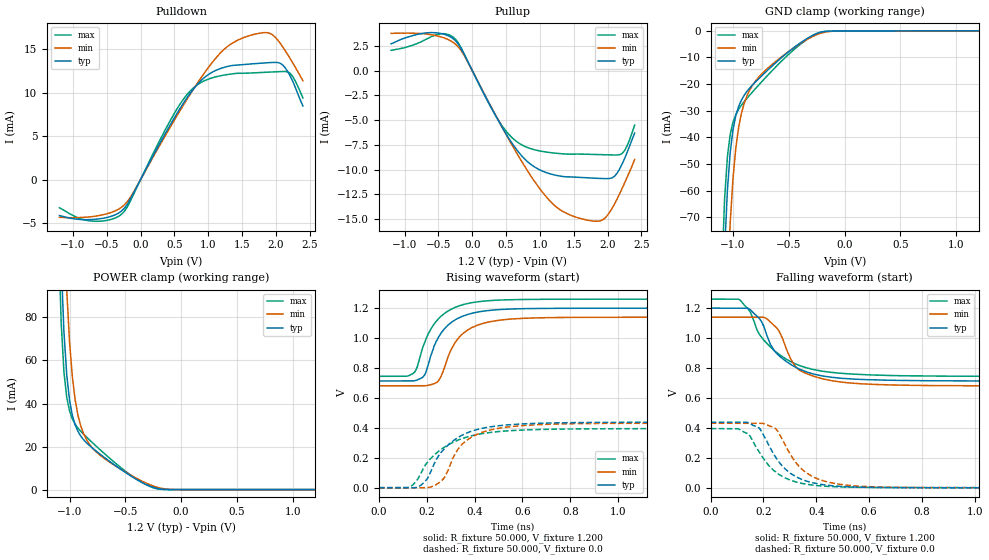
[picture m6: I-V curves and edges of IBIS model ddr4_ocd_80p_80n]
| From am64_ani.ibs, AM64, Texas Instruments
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|   Model ddr4_ocd_80p_80n
[Model] ddr4_ocd_80p_80n
Model_type I/O
Polarity   Non-Inverting
Enable   Active-High
Vinl =  0.700V
Vinh =  0.900V
Vmeas =  0.600V
C_comp   2.607pF   2.588pF   2.639pF
[Model Spec]
Vinh   0.900V   0.820V   0.980V
Vinl   0.700V   0.620V   0.780V
Vmeas   0.600V   NA   NA
[Temperature Range]   25.000   0.125k   -40.000
[Voltage Range]   1.200V   1.140V   1.260V
[Pullup Reference]   1.200V   1.140V   1.260V
[Pulldown Reference]   0.0V   0.0V   0.0V
[C Comp Corner]
C_comp   2.588pF   2.639pF   2.607pF
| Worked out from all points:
|   slope of the pulldown table from 0 to 0.18 V, typ, clamps not added: 67.6 ohm
|   slope of the pullup table from 0 to 0.18 V, typ, clamps not added: 74.1 ohm
|   GND clamp passes 1 mA (typ) near -0.25 V on its own axis
|   POWER clamp passes 1 mA (typ) near -0.25 V on its own axis
|   rising waveform, R_fixture 50.000, V_fixture 1.200: 20-80 % time 96.8ps typ, 97.8ps min, 100ps max; typ from 0.714 V to 1.2 V
|   rising waveform, R_fixture 50.000, V_fixture 0.0: 20-80 % time 136ps typ, 115ps min, 158ps max; typ from 0.002 V to 0.44 V
|   falling waveform, R_fixture 50.000, V_fixture 1.200: 20-80 % time 121ps typ, 91.9ps min, 143ps max; typ from 1.2 V to 0.714 V
|   falling waveform, R_fixture 50.000, V_fixture 0.0: 20-80 % time 110ps typ, 110ps min, 109ps max; typ from 0.44 V to 0.002 V
[Pulldown]
|Voltage   I(typ)   I(min)   I(max)
-1.2V     -4.138mA   -4.341mA   -3.244mA
-755mV    -4.611mA   -4.296mA   -4.748mA
-309mV    -3.777mA   -3.332mA   -4.155mA
-124mV    -1.85mA    -1.702mA   -2.032mA
396mV     5.718mA    5.465mA    6.181mA
693mV     9.481mA    9.32mA     9.848mA
990mV     12.02mA    12.77mA    11.53mA
1.398V    13.17mA    15.89mA    12.21mA
1.843V    13.43mA    16.92mA    12.35mA
2.066V    13.39mA    15.67mA    12.43mA
2.214V    11.88mA    13.89mA    12.21mA
2.4V      8.473mA    11.38mA    9.385mA
[Pullup]
|Voltage   I(typ)   I(min)   I(max)
-1.2V     2.716mA    3.765mA    2.056mA
-606mV    3.849mA    3.636mA    3.437mA
-421mV    3.694mA    3.326mA    3.74mA
-235mV    2.926mA    2.597mA    3.08mA
285mV     -3.787mA   -3.737mA   -3.812mA
544mV     -6.885mA   -6.995mA   -6.474mA
915mV     -9.714mA   -11.15mA   -7.988mA
1.361V    -10.72mA   -14.32mA   -8.419mA
1.955V    -10.91mA   -14.94mA   -8.5mA
2.103V    -10.67mA   -13.48mA   -8.524mA
2.214V    -9.447mA   -11.91mA   -8.38mA
2.4V      -6.303mA   -8.979mA   -5.506mA
[GND_clamp]
|Voltage   I(typ)   I(min)   I(max)
-1.2V     -396.3mA   -450.8mA   -370.5mA
-1.1V     -118.3mA   -172.8mA   -91.44mA
-1.075V   -83.02mA   -129.3mA   -63.08mA
-1.05V    -59.94mA   -96.19mA   -47.32mA
-1.025V   -45.76mA   -72.24mA   -38.96mA
-1V       -37.22mA   -55.56mA   -34.32mA
-975mV    -31.95mA   -44.18mA   -31.47mA
-925mV    -26.07mA   -31.12mA   -27.96mA
-775mV    -18.22mA   -17.64mA   -20.64mA
-425mV    -5.392mA   -5.54mA    -6.048mA
-175mV    -232.3uA   -493.9uA   -237.3uA
1.2V      0A         0A         0A
[POWER_clamp]
|Voltage   I(typ)   I(min)   I(max)
-1.2V     594.8mA    732.7mA    623.3mA
-1.1V     157.8mA    248.4mA    121.5mA
-1.075V   106.2mA    179.2mA    77.8mA
-1.05V    73.23mA    128.5mA    54.67mA
-1.025V   53.34mA    92.89mA    42.85mA
-1V       41.61mA    68.72mA    36.57mA
-975mV    34.56mA    52.6mA     32.87mA
-925mV    27.12mA    34.66mA    28.61mA
-825mV    20.64mA    21.33mA    23.28mA
-675mV    14.44mA    14mA       16.16mA
-200mV    388.1uA    876.1uA    237.2uA
1.2V      0A         0A         0A
[Ramp]
| variable   typ   min   max
dV/dt_r   0.262/0.136n   0.289/0.129n   0.236/0.159n
dV/dt_f   0.291/0.121n   0.306/0.107n   0.309/0.142n
R_load = 60.000
[Rising Waveform]
R_fixture= 50.000
V_fixture= 1.200
V_fixture_min= 1.140
V_fixture_max= 1.260
|time   V(typ)   V(min)   V(max)
0s        714.4mV    682.1mV    745.5mV
114ps     714.4mV    682.1mV    745.4mV
150ps     716.3mV    682.1mV    773.5mV
194ps     762.5mV    682.4mV    982.3mV
240ps     979.2mV    702.9mV    1.113V
278ps     1.07V      822.6mV    1.17V
325ps     1.127V     985.9mV    1.209V
426ps     1.177V     1.094V     1.245V
737ps     1.199V     1.137V     1.259V
3ns       1.2V       1.14V      1.26V
[Rising Waveform]
R_fixture= 50.000
V_fixture= 0.0
V_fixture_min= 0.0
V_fixture_max= 0.0
|time   V(typ)   V(min)   V(max)
0s        2.274mV    2.518mV    3.976mV
137ps     2.164mV    2.506mV    15.9mV
190ps     39.47mV    2.468mV    143.2mV
233ps     168.8mV    18.16mV    223.9mV
275ps     265.6mV    73.06mV    274.9mV
318ps     324.9mV    228.3mV    311.7mV
358ps     361.2mV    307.9mV    335.9mV
518ps     419.2mV    403.6mV    379.9mV
911ps     438.3mV    431.4mV    395.8mV
3ns       439.6mV    433mV      397.1mV
[Falling Waveform]
R_fixture= 50.000
V_fixture= 1.200
V_fixture_min= 1.140
V_fixture_max= 1.260
|time   V(typ)   V(min)   V(max)
0s        1.2V       1.14V      1.26V
112ps     1.2V       1.14V      1.253V
147ps     1.194V     1.14V      1.183V
176ps     1.145V     1.14V      1.053V
204ps     1.064V     1.138V     981.6mV
238ps     921.5mV    1.087V     921.5mV
262ps     877.3mV    1.038V     887.8mV
330ps     798.6mV    794.3mV    821.7mV
468ps     737mV      713.5mV    769.6mV
3ns       714.4mV    682mV      745.5mV
[Falling Waveform]
R_fixture= 50.000
V_fixture= 0.0
V_fixture_min= 0.0
V_fixture_max= 0.0
|time   V(typ)   V(min)   V(max)
0s        439.5mV    433mV      397.1mV
102ps     439.5mV    433mV      397.4mV
143ps     436.1mV    433mV      362.2mV
187ps     395.5mV    433.2mV    232.1mV
239ps     225.7mV    405.3mV    118.1mV
281ps     129.5mV    291.9mV    69.2mV
343ps     59.86mV    130mV      32.84mV
471ps     14.57mV    30.87mV    9.765mV
783ps     3.072mV    4.082mV    4.339mV
3ns       2.273mV    2.51mV     3.975mV
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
